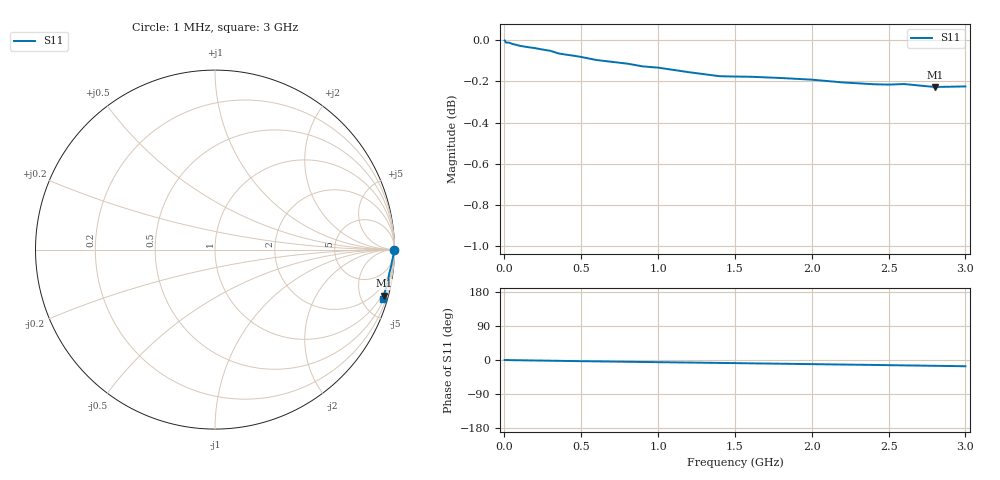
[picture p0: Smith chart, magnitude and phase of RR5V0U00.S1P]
! SIEMENS Small Signal Semiconductors
! BA595
! Si PIN Diode in SOD323
! VR = 5 V
! S-Parameters:  July  1992
# GHz  S  MA  R  50
!  f  S11
! GHz  MAG  ANG
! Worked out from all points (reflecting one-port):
!   33 points, 1 MHz to 3 GHz, reference 50 ohm
!   lowest |S11| = -0.2 dB at 2.8 GHz (marker M1), VSWR 76.52, Z = 36.5 - j369 ohm
!   phase of S11 starts at 0 deg and turns -16 deg over the sweep
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0.001  0.9999 0.0
0.003  0.9997 0.0
0.01  0.9987 -0.1
0.03  0.9987 -0.3
0.05  0.998 -0.4
0.06  0.9978 -0.5
0.1  0.9969 -0.7
0.3  0.9941 -1.9
0.35  0.9927 -2.2
0.4  0.992 -2.5
0.5  0.9907 -3.1
0.6  0.989 -3.6
0.7  0.988 -4.1
0.8  0.987 -4.7
0.9  0.9855 -5.2
1  0.9848 -5.7
1.2  0.9823 -6.7
1.4  0.9801 -7.7
1.5  0.9799 -8.2
1.6  0.9798 -8.8
1.8  0.9791 -9.8
2  0.9782 -10.9
2.2  0.9767 -12.0
2.4  0.9757 -13.0
2.5  0.9755 -13.6
2.6  0.9758 -14.2
2.8  0.9742 -15.3
3  0.9745 -16.5
